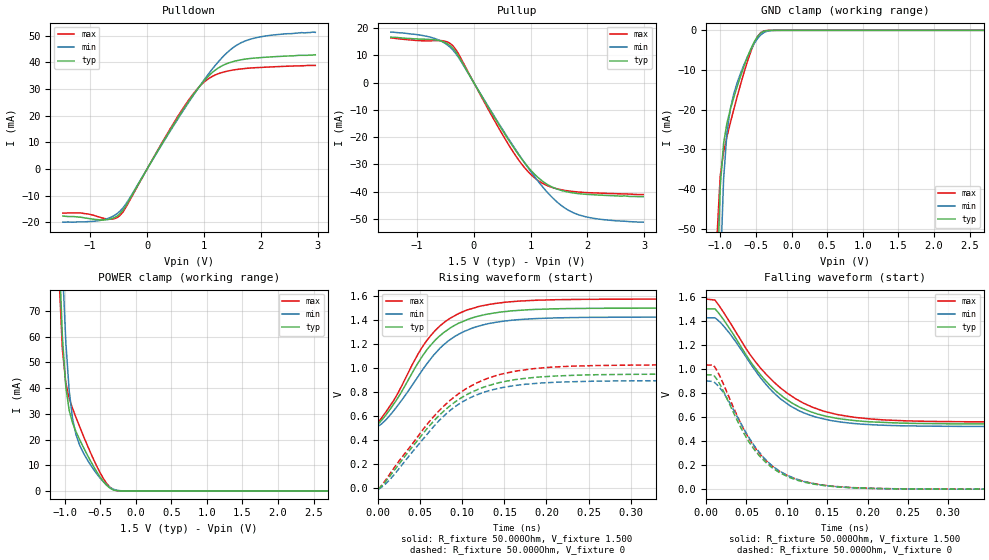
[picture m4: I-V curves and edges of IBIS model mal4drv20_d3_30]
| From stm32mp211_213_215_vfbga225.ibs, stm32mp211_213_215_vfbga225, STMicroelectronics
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[Model] mal4drv20_d3_30
Model_type   I/O
Polarity   Non-Inverting
Enable   Active-High
C_comp   1.836pF   1.830pF   1.844pF
C_comp_pullup   929.639fF   923.197fF   937.397fF
C_comp_pulldown 781.611fF   776.676fF   790.636fF
Vinh = 885.000mV
Vinl = 615.000mV
Vmeas = 750.000mV
Vref = 750.000mV
Rref = 50Ohms
Cref = 0pF
[Model Spec]
Vinh   885.000mV   848.000mV   923.000mV
Vinl   615.000mV   578.000mV   653.000mV
Vmeas   750.000mV   713.000mV   788.000mV
Vref   750.000mV   713.000mV   788.000mV
D_overshoot_ampl_h 0.4 NA   NA
D_overshoot_ampl_l 0.4 NA   NA
D_overshoot_area_l 100.000m NA   NA
D_overshoot_area_h 100.000m NA   NA
[Receiver Thresholds]
Vth = 750.000mV
Vth_min = 713.000mV
Vth_max = 788.000mV
Vinh_ac = 135.000mV
Vinh_dc = 100.000mV
Vinl_ac = -135.000mV
Vinl_dc = -100.000mV
Tslew_ac = 5.000ns
Threshold_sensitivity = 0.5
Reference_supply Pullup_ref
[Temperature Range]   25.000   125.000   -40.000
[Voltage Range]   1.500V   1.425V   1.575V
[GND Clamp Reference]   0.00V   0.00V   0.00V
[C Comp Corner]
| variable   typ   min   max
C_comp 1.844pF   1.836pF   1.830pF
C_comp_pullup 929.639fF   937.397fF   923.197fF
C_comp_pulldown 776.676fF   790.636fF   781.611fF
[Pulldown Reference]   0.00V   0.00V   0.00V
[POWER Clamp Reference]   1.500V   1.425V   1.575V
[Pullup Reference]   1.500V   1.425V   1.575V
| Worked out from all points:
|   slope of the pulldown table from 0 to 0.225 V, typ, clamps not added: 27.6 ohm
|   slope of the pullup table from 0 to 0.225 V, typ, clamps not added: 28.2 ohm
|   GND clamp passes 1 mA (typ) near -0.45 V on its own axis
|   POWER clamp passes 1 mA (typ) near -0.36 V on its own axis
|   rising waveform, R_fixture 50.000Ohm, V_fixture 1.500: 20-80 % time 58.6ps typ, 62.4ps min, 56.1ps max; typ from 0.538 V to 1.5 V
|   rising waveform, R_fixture 50.000Ohm, V_fixture 0: 20-80 % time 77.2ps typ, 73.2ps min, 80.7ps max; typ from -0.001 V to 0.951 V
|   falling waveform, R_fixture 50.000Ohm, V_fixture 1.500: 20-80 % time 70.7ps typ, 67.4ps min, 77.6ps max; typ from 1.5 V to 0.542 V
|   falling waveform, R_fixture 50.000Ohm, V_fixture 0: 20-80 % time 54.2ps typ, 55.8ps min, 54.7ps max; typ from 0.952 V to 0 V
[GND Clamp]
-1.48V    -1.637A    -1.644A    -1.658A
-1.05V    -67.86mA   -111.2mA   -53.06mA
-1.002V   -39.45mA   -62.21mA   -36.77mA
-954.6mV  -28.48mA   -37.5mA    -30.67mA
-906.8mV  -23.32mA   -25.75mA   -26.73mA
-859.1mV  -19.86mA   -19.72mA   -23.25mA
-763.6mV  -14.17mA   -13.2mA    -16.7mA
-668.2mV  -9.09mA    -8.668mA   -10.65mA
-525mV    -2.932mA   -3.341mA   -3.236mA
-429.5mV  -625.7uA   -1.091mA   -535.7uA
-238.6mV  -2.309uA   -20.7uA    -473nA
2.959V    72.19nA    968.6nA    105nA
[Power Clamp]
-1.459V   654.6mA    675.2mA    655.4mA
-1.077V   94.79mA    129.9mA    83.6mA
-1.03V    59.92mA    88.13mA    55.16mA
-981.8mV  40.46mA    57.96mA    42.01mA
-934.1mV  31.26mA    38.88mA    36.03mA
-886.4mV  26.43mA    28.01mA    32.07mA
-838.6mV  23.06mA    21.89mA    28.58mA
-647.7mV  12.32mA    10.7mA     15.7mA
-504.6mV  5.603mA    5.163mA    7.311mA
-361.4mV  1.062mA    1.366mA    1.412mA
-218.2mV  16.86uA    87.94uA    13.19uA
2.98V     -71.2nA    -1.524uA   -71.42nA
[Pulldown]
-1.48V    -17.6mA    -19.9mA    -16.5mA
-1.145V   -18.1mA    -19.8mA    -16.5mA
-763.6mV  -19.05mA   -18.97mA   -18.45mA
-620.5mV  -18.58mA   -17.91mA   -18.76mA
-477.3mV  -16.72mA   -15.79mA   -17.42mA
-334.1mV  -12.35mA   -11.85mA   -12.88mA
620.5mV   21.76mA    21.37mA    22.35mA
906.8mV   30.5mA     30.49mA    30.58mA
1.145V    36.12mA    37.39mA    34.67mA
1.48V     40.04mA    44.92mA    36.97mA
1.766V    41.29mA    48.29mA    37.75mA
2.959V    42.8mA     51.2mA     38.8mA
[Pullup]
-1.459V   16.7mA     18.54mA    16.4mA
-743.2mV  15.8mA     16.57mA    15.36mA
-504.6mV  14.73mA    14.41mA    15.2mA
-361.4mV  12.47mA    11.83mA    13.39mA
-265.9mV  9.603mA    9.165mA    10.45mA
688.6mV   -23.47mA   -23.1mA    -25.33mA
927.3mV   -30.32mA   -30.45mA   -32.06mA
1.166V    -35.5mA    -37.13mA   -36.44mA
1.5V      -39.34mA   -44.47mA   -39.17mA
1.786V    -40.63mA   -48.1mA    -40.07mA
2.216V    -41.31mA   -50.16mA   -40.58mA
2.98V     -41.9mA    -51.26mA   -41.1mA
[Ramp]
R_load=50.000Ohm
dV/dt_r   572.670mV/69.000ps  540.058mV/68.500ps  613.140mV/68.500ps
dV/dt_f   572.670mV/63.500ps  540.058mV/63.000ps  613.140mV/67.000ps
[Rising waveform]
R_fixture=50.000Ohm
V_fixture=1.500
V_fixture_min=1.425
V_fixture_max=1.575
0s        538.1mV    516.6mV    552.6mV
10ps      618.3mV    576.1mV    644.6mV
20ps      716.7mV    659.9mV    749.7mV
46ps      1.028V     916.9mV    1.101V
60ps      1.172V     1.056V     1.251V
82ps      1.318V     1.22V      1.399V
106ps     1.405V     1.318V     1.485V
139ps     1.46V      1.381V     1.538V
191ps     1.49V      1.414V     1.566V
469ps     1.5V       1.425V     1.575V
[Rising waveform]
R_fixture=50.000Ohm
V_fixture=0
0s        -895.2uV   -4.196mV   -6.944mV
15ps      112mV      81.64mV    131.1mV
57ps      487.9mV    441mV      523.1mV
77ps      637mV      595.2mV    678.2mV
105ps     778.6mV    739mV      830.8mV
122ps     833.3mV    791.5mV    892.3mV
144ps     880mV      833.7mV    946.7mV
180ps     919mV      869.1mV    992.4mV
235ps     941.6mV    888.6mV    1.018V
470ps     950.8mV    896.4mV    1.028V
[Falling waveform]
R_fixture=50.000Ohm
V_fixture=1.500
V_fixture_min=1.425
V_fixture_max=1.575
0s        1.5V       1.426V     1.582V
11ps      1.5V       1.426V     1.574V
19ps      1.435V     1.378V     1.498V
55ps      1.062V     1.044V     1.115V
85ps      825mV      794.9mV    884.9mV
115ps     685.1mV    652.9mV    736.6mV
146ps     611.5mV    583.6mV    648.4mV
182ps     571.6mV    547mV      599mV
244ps     549.2mV    527.4mV    569.2mV
480ps     542mV      521.3mV    559.2mV
[Falling waveform]
R_fixture=50.000Ohm
V_fixture=0
0s        951.6mV    900.8mV    1.033V
9ps       951.6mV    895.9mV    1.033V
12ps      926.5mV    878.8mV    1.003V
25ps      766.3mV    766.5mV    818.9mV
45ps      486.7mV    523mV      519.6mV
66ps      277.5mV    305.9mV    296.9mV
89ps      145.7mV    158.8mV    156.9mV
116ps     68.53mV    74.64mV    74.18mV
206ps     6.028mV    6.24mV     6.679mV
478ps     5.333uV    13.56uV    5.449uV
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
